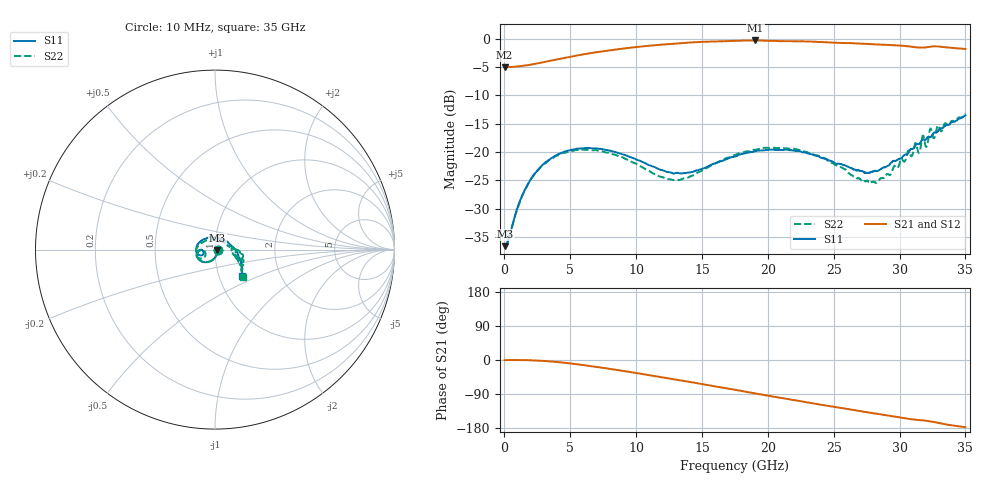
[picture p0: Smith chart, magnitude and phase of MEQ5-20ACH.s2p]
! MARKI MICROWAVE INC.
! Email:  support@markimicrowave.com  Phone:  408-778-4200
! Model Number:  MEQ5-20ACH  Date:  6/18
! Filename:		MEQ5-20ACH.S2P  Version: 1.0
! Description:  2-port S-parameter data for chip equalizer
! Features:		Low Insertion Loss, Excellent Return Loss
! Frequency Measured: 	10 MHz to 35 GHz
!S2P File: Measurements: S11, S21, S12, S22:
# Hz S  dB  R 50
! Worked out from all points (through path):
!   1601 points, 10 MHz to 35 GHz, reference 50 ohm
!   highest |S21| = -0.29 dB at 19.04 GHz (marker M1); lowest = -5.1 dB at 10 MHz (marker M2)
!   group delay of S21, straight-line fit = 15.4 ps
!   lowest |S11| = -36.7 dB at 53.74 MHz (marker M3), VSWR 1.03, Z = 51.4 - j0.503 ohm
!   |S11| at or under -10 dB: start of sweep to end of sweep
!   |S22| runs from -36.6 to -13.2 dB; largest |S21 - S12| = 0.0082
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1e7  -36.56 -19.0  -5.06 -0.3  -5.11 -0.3  -36.61 -5.2
5.37375e7  -36.65 -19.4  -5.05 -0.3  -5.08 -0.3  -36.62 -7.9
1.256519e9  -28.20 -84.8  -4.82 -0.1  -4.82 -0.1  -28.25 -84.4
2.306219e9  -23.81 -107.4  -4.43 -1.1  -4.43 -1.1  -23.86 -107.4
3.880769e9  -20.66 -130.9  -3.69 -4.9  -3.70 -4.9  -20.72 -130.6
5.848956e9  -19.36 -153.0  -2.80 -12.8  -2.80 -12.7  -19.60 -152.9
8.429469e9  -20.03 -172.9  -1.90 -25.6  -1.90 -25.6  -20.51 -172.4
1.168791e10  -22.98 -177.9  -1.09 -43.8  -1.08 -43.8  -24.25 -172.6
1.337181e10  -23.80 -167.0  -0.78 -53.6  -0.78 -53.7  -24.90 -156.9
1.7505e10  -20.78 -160.0  -0.36 -78.6  -0.37 -78.8  -20.54 -147.6
1.903581e10  -19.87 -168.0  -0.29 -88.3  -0.30 -88.1  -19.62 -155.5
2.334396e10  -20.43 155.0  -0.51 -114.0  -0.50 -113.8  -20.36 167.8
2.725846e10  -23.56 86.1  -0.87 -136.3  -0.88 -136.0  -25.17 98.5
2.822069e10  -23.39 62.3  -1.01 -141.6  -0.95 -141.4  -25.44 66.7
2.918291e10  -22.39 37.8  -1.09 -146.6  -1.08 -147.0  -23.96 40.8
3.117297e10  -19.00 1.6  -1.49 -157.4  -1.53 -157.2  -18.53 -6.0
3.147913e10  -18.61 -5.2  -1.53 -158.6  -1.56 -158.3  -20.12 -7.7
3.176342e10  -17.78 -10.8  -1.56 -159.3  -1.56 -159.0  -17.11 -9.9
3.204772e10  -17.64 -13.2  -1.50 -160.5  -1.48 -160.1  -19.09 -11.3
3.235388e10  -17.37 -18.6  -1.39 -161.9  -1.34 -161.7  -15.85 -14.2
3.261631e10  -16.57 -20.2  -1.33 -163.8  -1.32 -163.7  -17.55 -17.9
3.5e10  -13.53 -43.8  -1.80 -177.3  -1.78 -177.1  -13.21 -44.4
